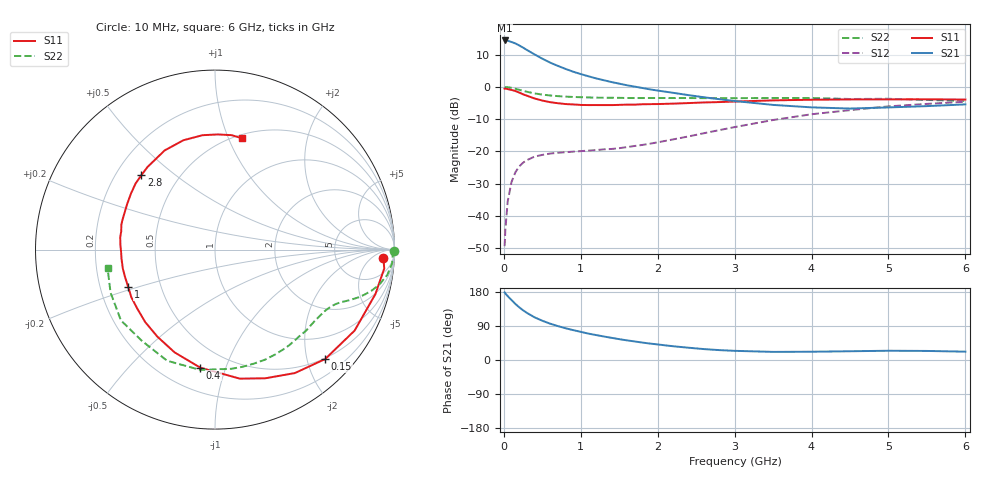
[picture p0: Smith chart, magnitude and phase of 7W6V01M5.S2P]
! Infineon Technologies  Discrete & RF Semiconductors
! BFS17W
! Si NPN RF Bipolar Junction Transistor in SOT323
! VCE = 6 V  IC = 1.5 mA
! Common Emitter S-Parameters:  August  1999
# GHz  S  MA  R  50
!  f  S11  S21  S12  S22
! GHz  MAG  ANG  MAG  ANG  MAG  ANG  MAG  ANG
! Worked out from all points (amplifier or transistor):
!   36 points, 10 MHz to 6 GHz, reference 50 ohm
!   highest |S21| = 14.4 dB at 10 MHz (marker M1)
!   |S21| within 3 dB of that: start of sweep to 303.3 MHz
!   unconditionally stable (mu >= 1): 938.6 MHz to 3.145 GHz; 4.086 GHz to end of sweep
!   at 250 MHz: K = 0.31, MSG = 17.8 dB, |S12| = -23.5 dB
!   at 1.4 GHz: K = 1.28, MAG = 7.2 dB, |S12| = -19.2 dB
!   at 6 GHz: K = 1.08, MAG = -2.2 dB, |S12| = -4.6 dB
!   S11 on the Smith chart (normalised r, x): 10 MHz: 19, -16; 150 MHz: 0.48, -2.34; 400 MHz: 0.35, -0.82; 1 GHz: 0.32, -0.19; 2.8 GHz: 0.31, +0.38; 6 GHz: 0.54, +1.12
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0.01  0.94 -3.0  5.265 178.4  0.0034 84.9  0.9999 -0.4
0.02  0.9487 -6.4  5.259 175.5  0.0062 85.2  0.9909 -1.7
0.05  0.9274 -15.5  5.211 168.6  0.0168 83.8  0.9897 -4.4
0.1  0.8993 -30.1  4.98 158.2  0.0337 74.2  0.9703 -8.4
0.15  0.8652 -44.8  4.734 147.9  0.0475 66.1  0.9369 -11.9
0.2  0.8193 -57.1  4.409 139.1  0.0586 60.0  0.9045 -14.5
0.25  0.77 -68.6  4.075 131.2  0.067 54.2  0.8709 -16.7
0.3  0.7322 -79.1  3.747 124.3  0.0734 50.9  0.8428 -18.4
0.4  0.6629 -97.1  3.195 112.6  0.0833 44.5  0.7951 -20.9
0.5  0.6152 -111.5  2.748 103.6  0.0885 41.3  0.7614 -22.6
0.6  0.5816 -123.5  2.392 96.0  0.0927 39.3  0.7387 -24.2
0.7  0.5606 -133.9  2.129 89.6  0.0954 38.6  0.7218 -25.9
0.8  0.5438 -142.7  1.91 83.9  0.0973 38.4  0.7092 -27.7
1  0.5265 -156.7  1.584 74.3  0.1011 40.3  0.6943 -31.2
1.1  0.524 -163.4  1.465 69.6  0.1033 41.4  0.6881 -33.4
1.6  0.5326 172.5  1.063 51.8  0.1169 51.5  0.6742 -44.7
2.2  0.5518 152.3  0.812 36.3  0.1538 63.4  0.6738 -60.1
2.8  0.5833 134.6  0.647 26.1  0.2142 68.0  0.6707 -76.9
3.5  0.6197 116.9  0.527 21.4  0.3076 65.8  0.6754 -97.0
4.5  0.6412 96.2  0.463 23.1  0.4372 53.8  0.6515 -128.7
5.5  0.6442 81.7  0.505 23.9  0.5471 40.2  0.6294 -157.6
6  0.6382 76.4  0.537 22.0  0.5895 33.8  0.6073 -170.4
